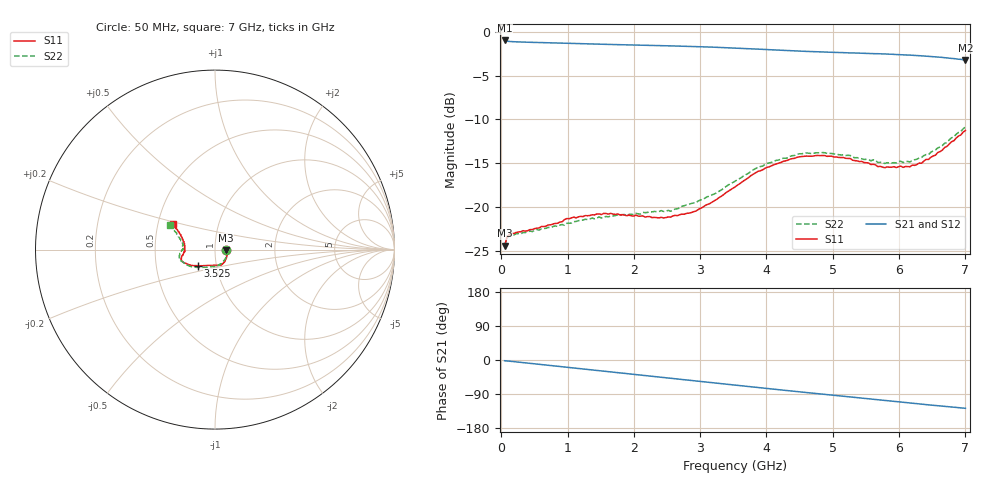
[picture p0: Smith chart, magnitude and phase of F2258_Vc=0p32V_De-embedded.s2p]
! Integrated Device Technology
! Corporate Headquarters
! 6024 Silver Creek Valley Road
! San Jose, CA 95138  USA
! Phone:  1-408-284-8200
! Toll Free:  1-800-223-1366
! Webpage:  http://www.idt.com/
! Timing and RF Division
! 515 Groton Road, Suite 102
! Westford, MA 01886-6024
! Device:  F2258
! Description: Voltage Variable RF Attenuator
! Frequency:  50.0 -  6000.00 MHz
! Package:  3x3 mm Thin QFN Plastic Package: 16 pin
! Ports:  2 RF, 2 DC
!  Pin  1  = NC
!  Pin  2  = NC
!  Pin  3  = RF2  = Port 2
!  Pin  4  = GND
!  Pin  5  = Vdd
!  Pin  6  = NC
!  Pin  7  = VCTRL
!  Pin  8  = NC
!  Pin  9  = GND
!  Pin 10  = RF1  = Port 1
!  Pin 11  = NC
!  Pin 12  = NC
!  Pin 13  = NC
!  Pin 14  = NC
!  Pin 15  = NC
!  Pin 16  = NC
! Vcntrl:  0.320 Volts
! Vdd:  +3.300 Volts
! Current:  1.088 mA
! Data:  The device was measured on a the F2258 evaluation board which has
!  individual transmission lines to the RF pins.  Data was collected
!  using a calibrated network analyzer.  The evaluation board was
!  de-embedded using a TRL calibration technique.
!  The reference plane is the edge of the package pin.
! Misc:  SN 10
!  Action Tracker AT0285
! Date Measured:  2014-12-10
! Date:  2016-01-13  MJV
! Note:
!  Integrated Device Technology supplies this data as a sample of measured
!  data at the package pin for this product.  Your particular data for this
!  product may vary.
!  Data was taken at 25 degrees C.
!  Integrated Device Technology reserves the right to change this data at anytime.
!Freq_(GHz)  S11M_(dB)  S11P_(deg)  S21M_(dB)  S21P_(deg)  S12M_(dB)  S12P_(deg)  S22M_(dB)  S22P_(deg)
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# GHz S dB R 50
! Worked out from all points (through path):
!   201 points, 50 MHz to 7 GHz, reference 50 ohm
!   highest |S21| = -0.98 dB at 50 MHz (marker M1); lowest = -3.2 dB at 7 GHz (marker M2)
!   group delay of S21, straight-line fit = 50.5 ps
!   lowest |S11| = -24.4 dB at 50 MHz (marker M3), VSWR 1.13, Z = 56.4 - j0.4 ohm
!   |S11| at or under -10 dB: start of sweep to end of sweep
!   |S22| runs from -24.5 to -10.9 dB; largest |S21 - S12| = 0.00038
!   S11 on the Smith chart (normalised r, x): 50 MHz: 1.13, -0.01; 3.525 GHz: 0.82, -0.15; 7 GHz: 0.60, +0.19
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0.05  -24.44 -3.4  -0.98 -1.9  -0.98 -1.9  -24.49 -3.0
0.08475  -23.49 -5.7  -1.06 -2.5  -1.06 -2.5  -23.57 -5.3
0.15425  -23.01 -8.9  -1.11 -3.6  -1.12 -3.6  -23.20 -9.2
0.71025  -22.06 -36.0  -1.25 -14.1  -1.25 -14.1  -22.35 -37.9
0.98825  -21.34 -49.6  -1.30 -19.3  -1.30 -19.3  -21.88 -53.8
1.2315  -21.12 -57.8  -1.36 -23.8  -1.36 -23.8  -21.52 -62.8
1.6485  -20.74 -69.3  -1.44 -31.4  -1.44 -31.4  -21.05 -75.8
2.37825  -21.26 -90.4  -1.57 -44.8  -1.57 -44.8  -20.53 -93.6
2.552  -21.18 -96.3  -1.60 -48.0  -1.60 -48.0  -20.50 -98.8
2.93425  -20.48 -113.0  -1.68 -55.1  -1.68 -55.1  -19.53 -112.3
3.525  -17.72 -136.3  -1.85 -66.2  -1.85 -66.2  -17.08 -135.1
4.0115  -15.48 -150.2  -2.03 -75.2  -2.03 -75.2  -15.03 -150.6
4.46325  -14.33 -158.8  -2.19 -83.4  -2.19 -83.4  -13.99 -161.7
4.7065  -14.20 -162.1  -2.26 -87.7  -2.26 -87.7  -13.89 -166.0
5.15825  -14.36 -167.5  -2.38 -95.6  -2.39 -95.6  -14.06 -172.9
5.64475  -15.21 -175.6  -2.50 -104.0  -2.50 -104.0  -14.68 -179.3
5.6795  -15.41 -175.7  -2.50 -104.6  -2.50 -104.6  -14.93 -179.5
5.85325  -15.47 -179.8  -2.55 -107.8  -2.56 -107.8  -14.96 175.9
6.166  -15.41 172.3  -2.66 -113.4  -2.66 -113.4  -14.88 169.9
6.33975  -15.01 165.9  -2.74 -116.5  -2.74 -116.5  -14.35 165.5
6.722  -13.09 154.0  -2.98 -123.1  -2.98 -123.1  -12.65 156.4
7  -11.27 148.5  -3.22 -127.4  -3.22 -127.4  -10.87 151.5
